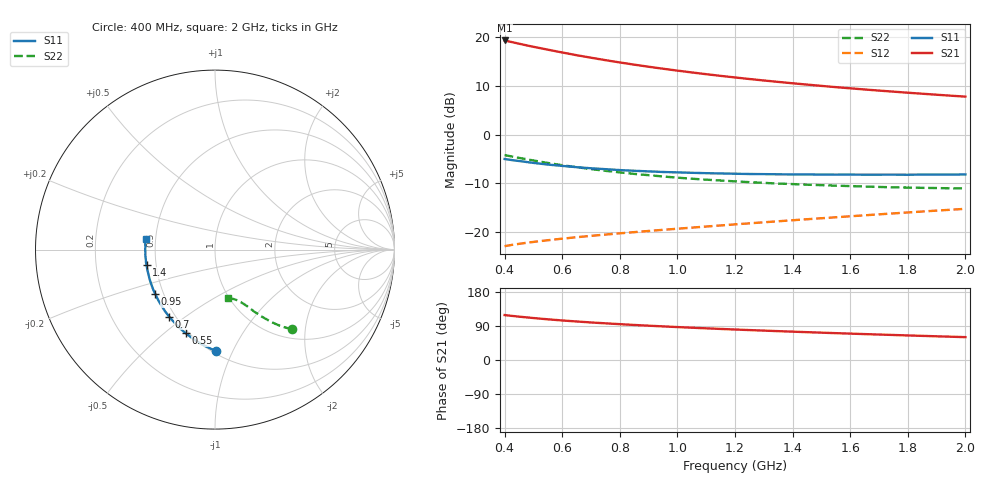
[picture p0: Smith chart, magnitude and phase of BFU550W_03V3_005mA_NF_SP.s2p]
! Filename:  P:\Prog\Test\Noise\ATS_data\Testdata_Net\06 Compressed Noise after Statistics\BFU550W_APM2013_11_D05_03p3V_005mA_NF_CM01_D.sf
! Date/Time: Tue 26/Mar/2013 16:25:27
! BFU550W_APM2013_11_D05_03p3V_1to35mA_NF_CM01_Bias4_R.sf
! Noise Parameter Data File
! BFU550W_APM2013_11_D05_03p3V_1to35mA_NF_CM01
! Date/time: Mon Mar 25 12:16:07 2013
! VAR V_out= 3.300000
! VAR I_out= 4.995000
! VAR V_in= 0.814600
! VAR I_in= 0.052405
! Device data file deembeded for feedlines and parallel
! Original file: \06 Compressed Noise after Statistics\BFU550W_APM2013_11_D05_03p3V_005mA_NF_CM01_R.sf
! Feed-files: PR019V01_070313_Feed1.s2p, PR019V01_070313_Feed2.s2p
! Parallel-file: PR019V01_070313_Par.s2p
# MHz S MA R 50
!  Freq-MHz  S11-mag  S11-arg  S21-mag  S21-arg  S12-mag  S12-arg  S22-mag  S22-arg
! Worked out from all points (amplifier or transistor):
!   37 points, 400 MHz to 2 GHz, reference 50 ohm
!   highest |S21| = 19.4 dB at 400 MHz (marker M1)
!   |S21| within 3 dB of that: start of sweep to 647.3 MHz
!   unconditionally stable (mu >= 1): 1.663 GHz to end of sweep
!   at 500 MHz: K = 0.53, MSG = 20.1 dB, |S12| = -22.0 dB
!   at 1.1 GHz: K = 0.87, MSG = 15.7 dB, |S12| = -18.9 dB
!   at 2 GHz: K = 1.02, MAG = 10.6 dB, |S12| = -15.2 dB
!   lowest NFmin = 0.55 dB at 440 MHz
!   S11 on the Smith chart (normalised r, x): 400 MHz: 0.52, -0.86; 550 MHz: 0.48, -0.59; 700 MHz: 0.46, -0.43; 950 MHz: 0.45, -0.27; 1.4 GHz: 0.44, -0.09; 2 GHz: 0.44, +0.06
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400  0.5635 -89.5  9.319 118.6  0.07157 53.5  0.6177 -45.9
420  0.5522 -92.6  9.037 116.8  0.07331 52.9  0.6019 -46.9
440  0.542 -95.4  8.766 115.2  0.07488 52.4  0.5863 -47.8
460  0.5326 -98.1  8.502 113.7  0.07633 52.0  0.5716 -48.7
500  0.5138 -103.3  8.02 110.7  0.07916 51.2  0.5443 -50.3
550  0.4939 -109.2  7.495 107.4  0.08236 50.7  0.5131 -52.0
600  0.4784 -114.8  7.012 104.3  0.08548 50.3  0.4862 -53.3
650  0.4641 -119.6  6.574 101.7  0.08848 50.1  0.4645 -54.5
700  0.4525 -124.4  6.194 99.1  0.09134 50.1  0.4438 -55.7
750  0.4429 -128.7  5.847 96.8  0.09417 50.2  0.4259 -56.6
800  0.4334 -132.8  5.537 94.6  0.09701 50.3  0.4106 -57.6
850  0.4263 -136.7  5.258 92.5  0.09975 50.5  0.396 -58.3
950  0.4142 -143.5  4.774 88.7  0.1053 51.1  0.3725 -59.8
1050  0.4063 -149.7  4.371 85.2  0.111 51.8  0.3533 -61.2
1150  0.4002 -155.5  4.03 82.0  0.1169 52.3  0.3385 -62.5
1200  0.3974 -157.9  3.883 80.5  0.1199 52.7  0.3319 -63.3
1300  0.3938 -162.8  3.614 77.5  0.1259 53.3  0.3202 -64.5
1400  0.391 -167.3  3.382 74.8  0.1322 53.9  0.3111 -65.8
1500  0.3896 -171.5  3.18 72.1  0.1386 54.4  0.3033 -67.3
1650  0.3884 -177.3  2.921 68.4  0.1486 55.0  0.2938 -69.4
1750  0.3889 179.3  2.774 66.0  0.1554 55.4  0.2882 -71.0
2000  0.391 171.1  2.466 60.3  0.1733 55.9  0.2799 -75.3
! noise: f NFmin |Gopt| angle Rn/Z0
400  0.5865  0.1709  43.36  0.0955
460  0.5977  0.1544  56.52  0.0916
600  0.6293  0.1747  62.36  0.0979
800  0.6669  0.1974  86.52  0.0857
1000  0.718  0.217  97.36  0.084
1200  0.789  0.245  112.6  0.0767
1400  0.8104  0.2354  130.8  0.0745
1600  0.8117  0.2771  143.9  0.0646
1800  0.8742  0.2964  158.6  0.0616
2000  0.895  0.3049  173.7  0.0641
